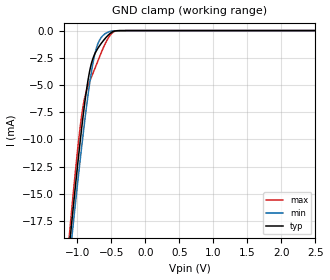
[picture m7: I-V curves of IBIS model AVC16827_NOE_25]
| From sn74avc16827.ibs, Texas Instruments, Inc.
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[Model]   AVC16827_NOE_25
Model_type  Input
Vinl=0.7
Vinh=1.7
| variable   typ   min   max
C_comp   2.47pF   1.68pF   2.81pF
[Temperature Range]   40   100   -40
| Ambient temperature   25   85   -40
[Voltage range]   2.5   2.3   2.7
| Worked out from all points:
|   GND clamp passes 1 mA (typ) near -0.62 V on its own axis
[GND Clamp]
| AVC16827_NOE_25
|   Voltage   I(typ)   I(min)   I(max)
-2.5V     -116.9mA   -113.2mA   -123.6mA
-1.11V    -19.59mA   -20.97mA   -18.51mA
-1.095V   -18.63mA   -20.05mA   -17.49mA
-1.065V   -16.75mA   -18.25mA   -15.49mA
-985mV    -11.89mA   -13.57mA   -10.49mA
-930mV    -8.788mA   -10.5mA    -7.655mA
-885mV    -6.49mA    -8.123mA   -6.066mA
-820mV    -3.852mA   -5.028mA   -4.756mA
-710mV    -1.78mA    -1.47mA    -3.027mA
-570mV    -594.8uA   -214.4uA   -983.4uA
-380mV    -6.887uA   -6.787uA   -6.353uA
2.5V      269.1pA    954.9pA    17.34pA
